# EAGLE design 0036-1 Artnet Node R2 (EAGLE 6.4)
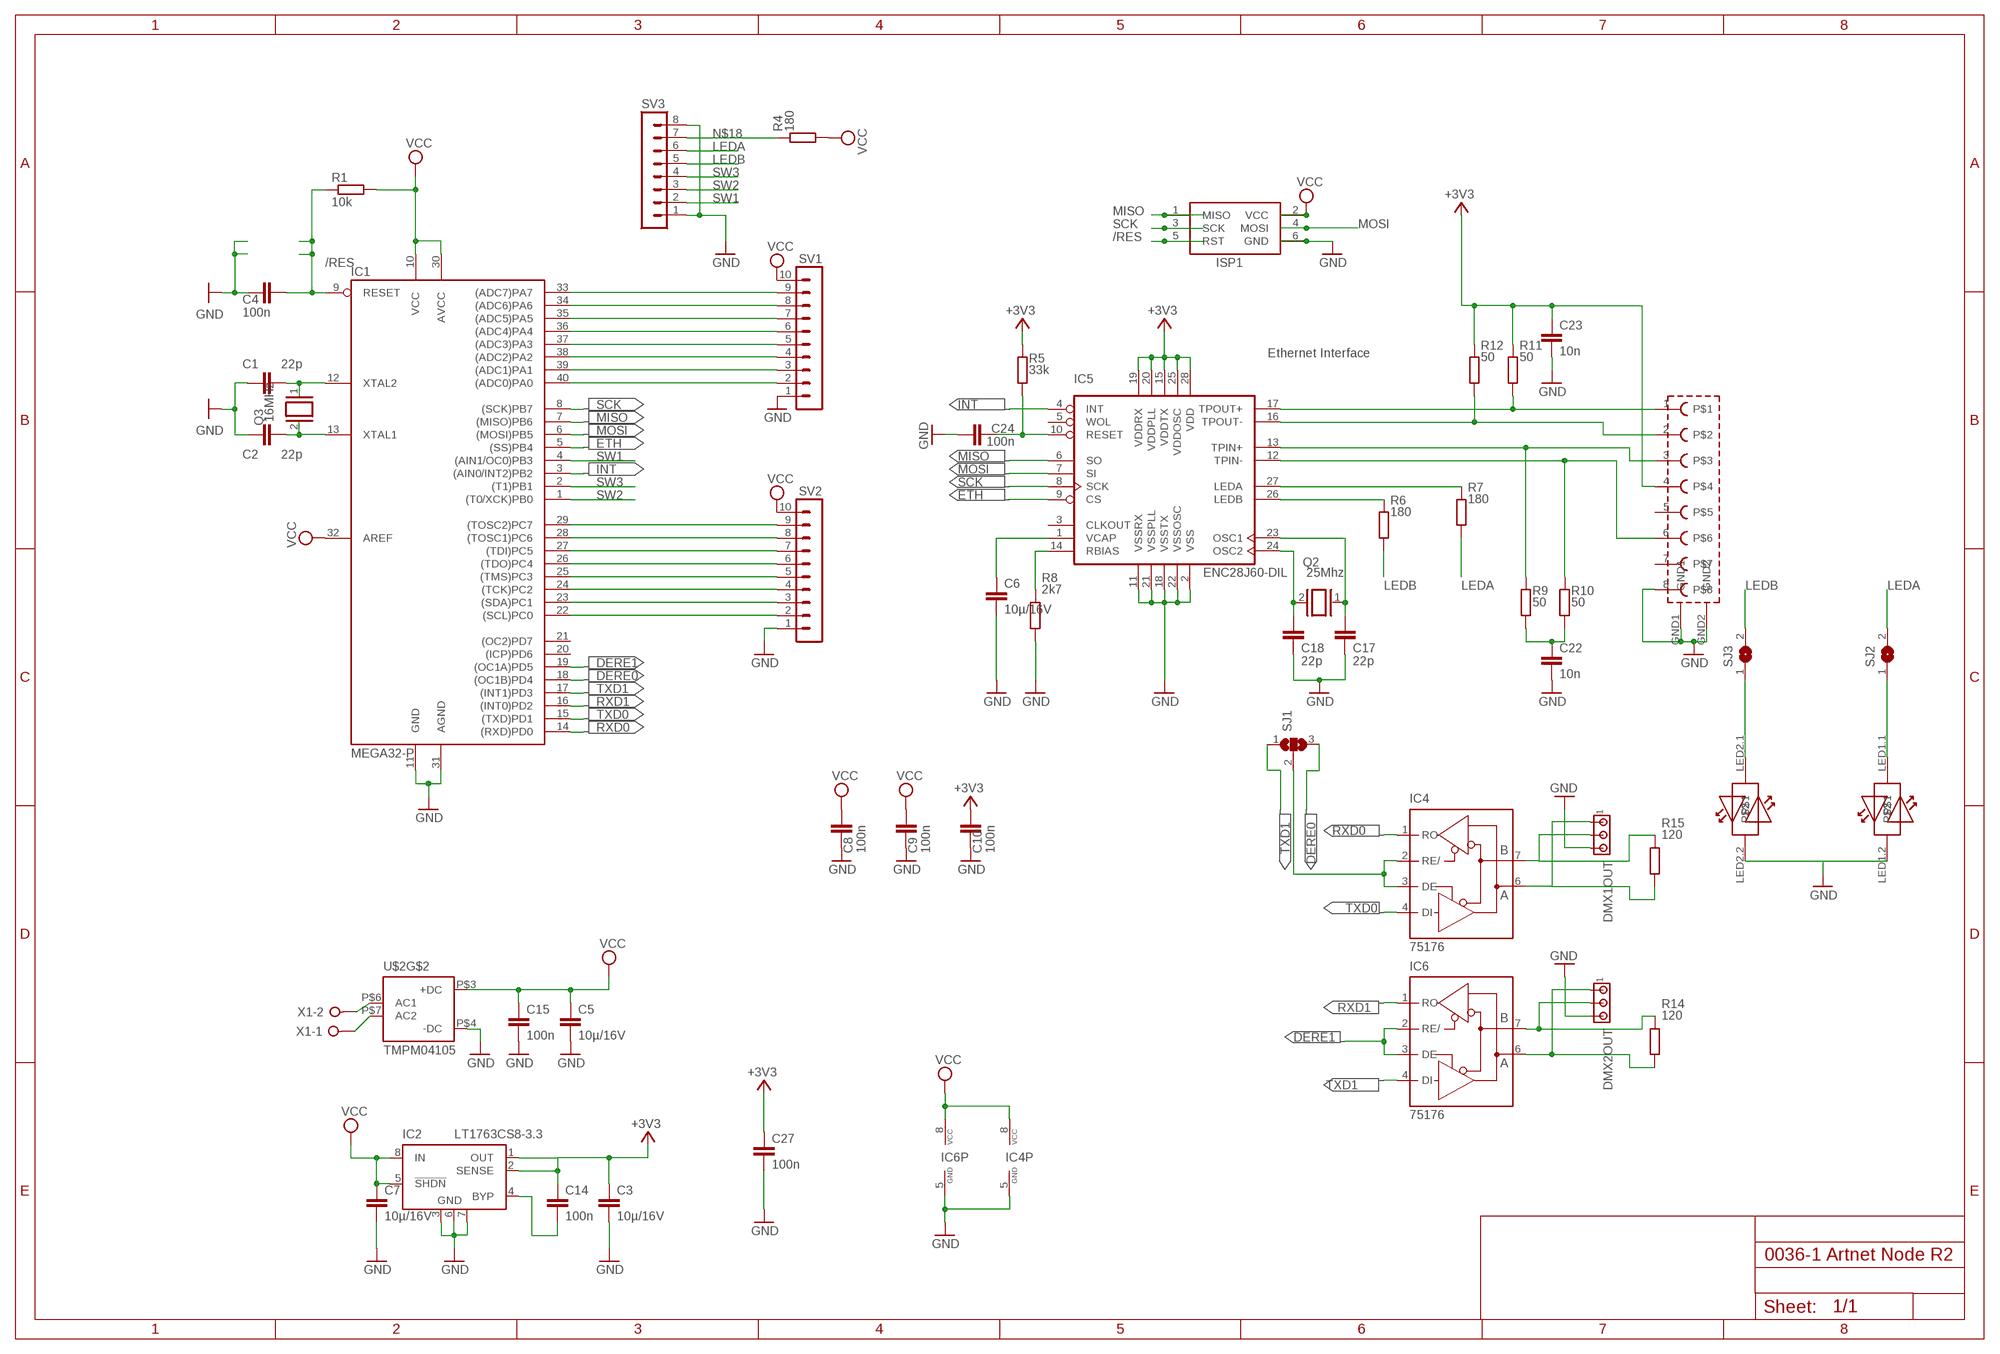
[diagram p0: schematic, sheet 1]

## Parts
C1  22p  C-EUC0805  [C0805]
C2  22p  C-EUC0805  [C0805]
C3  10µ/16V  C-EUC0805  [C0805]
C4  100n  C-EUC0805  [C0805]
C5  10µ/16V  C-EUC0805  [C0805]
C6  10µ/16V  C-EUC0805  [C0805]
C7  10µ/16V  C-EUC0805  [C0805]
C8  100n  C-EUC0805  [C0805]
C9  100n  C-EUC0805  [C0805]
C10  100n  C-EUC0805  [C0805]
C14  100n  C-EUC0805  [C0805]
C15  100n  C-EUC0805  [C0805]
C17  22p  C-EUC0805  [C0805]
C18  22p  C-EUC0805  [C0805]
C22  10n  C-EUC0805  [C0805]
C23  10n  C-EUC0805  [C0805]
C24  100n  C-EUC0805  [C0805]
C27  100n  C-EUC0805  [C0805]
DMX1OUT  MTA03-100  [10X03MTA]
DMX2OUT  MTA03-100  [10X03MTA]
IC1  MEGA32-P  [DIL40]
IC2  LT1763CS8-3.3  [SOIC8]
IC4  75176  MAX481CPA  [DIL08]
IC5  ENC28J60-DIL  [DIL28-3]
IC6  75176  MAX481CPA  [DIL08]
ISP1  AVRISP-6  [AVRISP]
Q2  25Mhz  XTAL/S  [QS]
Q3  16MHz  XTAL/S  [QS]
R1  10k  R-EU_R0805  [R0805]
R4  180  R-EU_R0805  [R0805]
R5  33k  R-EU_R0805  [R0805]
R6  180  R-EU_R0805  [R0805]
R7  180  R-EU_R0805  [R0805]
R8  2k7  R-EU_R0805  [R0805]
R9  50  R-EU_MELF0204W  [MINI_MELF-0204W]
R10  50  R-EU_MELF0204W  [MINI_MELF-0204W]
R11  50  R-EU_MELF0204W  [MINI_MELF-0204W]
R12  50  R-EU_MELF0204W  [MINI_MELF-0204W]
R14  120  R-EU_R0805  [R0805]
R15  120  R-EU_R0805  [R0805]
SJ1  SJ2W  [SJ_2]
SJ2  SJ  [SJ]
SJ3  SJ  [SJ]
SV1  MA10-1  [MA10-1]
SV2  MA10-1  [MA10-1]
SV3  MA08-1  [MA08-1]
U$1  MAGJACK  [MAGJACK]
U$2  TMPM04105  [4WSINGLE]
X1  W237-02P  [W237-132]

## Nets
+3V3: C3.1 C10.2 C14.1 C23.1 C27.1 IC2.1(OUT) IC2.2(SENSE) IC5.15(VDDTX) IC5.19(VDDRX) IC5.20(VDDPLL) IC5.25(VDDOSC) IC5.28(VDD) R5.2 R11.1 R12.1 U$1.4
/RES: C4.2 IC1.9(RESET) ISP1.5(RST) R1.1
DERE0: IC1.18((OC1B)PD4) SJ1.3
DERE1: IC1.19((OC1A)PD5) IC6.2(RE/) IC6.3(DE)
ETH: IC1.5((SS)PB4) IC5.9(CS)
GND: C1.1 C2.1 C3.2 C4.1 C5.2 C6.2 C7.2 C8.1 C9.1 C10.1 C15.2 C17.1 C18.1 C22.2 C23.2 C24.1 C27.2 DMX1OUT.3 DMX2OUT.3 IC1.11(GND) IC1.31(AGND) IC2.3(GND) IC2.6(GND) IC2.7(GND) IC4.5(GND) IC5.2(VSS) IC5.11(VSSRX) IC5.18(VSSTX) IC5.21(VSSPLL) IC5.22(VSSOSC) IC6.5(GND) ISP1.6(GND) R8.1 SV1.1 SV2.1 SV3.1 SV3.8 U$1.8 U$1.GND1 U$1.GND2 U$1.LED1.2 U$1.LED2.2 U$2.P$4(-DC)
INT: IC1.3((AIN0/INT2)PB2) IC5.4(INT)
LEDA: R7.1 SJ2.2 SV3.6
LEDB: R6.1 SJ3.2 SV3.5
MISO: IC1.7((MISO)PB6) IC5.6(SO) ISP1.1(MISO)
MOSI: IC1.6((MOSI)PB5) IC5.7(SI) ISP1.4(MOSI)
N$1: C2.2 IC1.13(XTAL1) Q3.2
N$2: C1.2 IC1.12(XTAL2) Q3.1
N$3: IC4.2(RE/) IC4.3(DE) SJ1.2
N$5: IC1.22((SCL)PC0) SV2.2
N$6: U$2.P$7(AC2) X1.1
N$7: U$2.P$6(AC1) X1.2
N$8: IC1.23((SDA)PC1) SV2.3
N$9: IC1.24((TCK)PC2) SV2.4
N$10: IC1.25((TMS)PC3) SV2.5
N$11: IC5.27(LEDA) R7.2
N$12: IC1.26((TDO)PC4) SV2.6
N$13: IC5.26(LEDB) R6.2
N$14: IC1.27((TDI)PC5) SV2.7
N$15: IC1.28((TOSC1)PC6) SV2.8
N$16: DMX2OUT.1 IC6.6(A) R14.1
N$17: DMX1OUT.1 IC4.6(A) R15.1
N$18: R4.2 SV3.7
N$19: IC1.29((TOSC2)PC7) SV2.9
N$20: C18.2 IC5.24(OSC2) Q2.2
N$21: C17.2 IC5.23(OSC1) Q2.1
N$22: IC5.12(TPIN-) R10.2 U$1.6
N$23: IC5.13(TPIN+) R9.2 U$1.3
N$24: IC5.16(TPOUT-) R12.2 U$1.2
N$25: IC5.17(TPOUT+) R11.2 U$1.1
N$26: IC5.14(RBIAS) R8.2
N$27: C6.1 IC5.1(VCAP)
N$28: SJ3.1 U$1.LED2.1
N$29: C22.1 R9.1 R10.1
N$30: C24.2 IC5.10(RESET) R5.1
N$31: DMX1OUT.2 IC4.7(B) R15.2
N$32: DMX2OUT.2 IC6.7(B) R14.2
N$33: SJ2.1 U$1.LED1.1
N$34: IC1.40((ADC0)PA0) SV1.2
N$35: C14.2 IC2.4(BYP)
N$36: IC1.39((ADC1)PA1) SV1.3
N$37: IC1.38((ADC2)PA2) SV1.4
N$38: IC1.37((ADC3)PA3) SV1.5
N$39: IC1.36((ADC4)PA4) SV1.6
N$40: IC1.35((ADC5)PA5) SV1.7
N$41: IC1.34((ADC6)PA6) SV1.8
N$42: IC1.33((ADC7)PA7) SV1.9
RXD0: IC1.14((RXD)PD0) IC4.1(RO)
RXD1: IC1.16((INT0)PD2) IC6.1(RO)
SCK: IC1.8((SCK)PB7) IC5.8(SCK) ISP1.3(SCK)
SW1: IC1.4((AIN1/OC0)PB3) SV3.2
SW2: IC1.1((T0/XCK)PB0) SV3.3
SW3: IC1.2((T1)PB1) SV3.4
TXD0: IC1.15((TXD)PD1) IC4.4(DI)
TXD1: IC1.17((INT1)PD3) IC6.4(DI) SJ1.1
VCC: C5.1 C7.1 C8.2 C9.2 C15.1 IC1.10(VCC) IC1.30(AVCC) IC1.32(AREF) IC2.5(!SHDN) IC2.8(IN) IC4.8(VCC) IC6.8(VCC) ISP1.2(VCC) R1.2 R4.1 SV1.10 SV2.10 U$2.P$3(+DC)
Unconnected: IC1.20((ICP)PD6) IC1.21((OC2)PD7) IC5.3(CLKOUT) IC5.5(WOL) U$1.5 U$1.7

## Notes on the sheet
- Ethernet Interface

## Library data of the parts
C1-C10 C14 C15 C17 C18 C22-C24 C27 = rcl:C-EU: CAPACITOR, European symbol
DMX1OUT DMX2OUT = con-amp:MTA03-100: AMP connector
IC1 = avr-1:MEGA32-P: MICROCONTROLLER 32 Kbytes FLASH 2 Kbytes SRAM 1 Kbytes EEPROM USART 8-channel 10 bit ADC
IC2 = linear-technology:LT1763CS8: 500mA, Low Noise, LDO Micropower Regulators Source: http://cds.linear.com/docs/Datasheet/1763ff.pdf; MPN: LT1763CS8-3.3; OC_FARNELL: 1273617; OC_NEWARK: 57M6055
IC4 IC6 = maxim:MAX481CPA: RS485 TRANSEIVER; MPN: MAX481CPA+; OC_FARNELL: unknown; OC_NEWARK: 99K3445
IC5 = enc28j60centered:ENC28J60-*: Microchip 10Mbit Ethernet controller with SPI interface Improved SOIC28 layout (pads in 0.01 raster, pin1 slightly smaller). Pin 6 (SO) changed from Out (paralleling several Outs gives an error) to OC. Author: Profi from mikrocontroller.net - forum Date: 2006.0827
ISP1 = adafruit:AVRISP: AVR ISP HEADER Standard 6 pin header for AVR programming
Q2 Q3 = special:XTAL/S: CRYSTAL
R1 R4-R12 R14 R15 = rcl:R-EU_: RESISTOR, European symbol
SJ1 = jumper:SJ2W: SMD solder JUMPER
SJ2 SJ3 = jumper:SJ: SMD solder JUMPER
SV1 SV2 = con-lstb:MA10-1: PIN HEADER; OC_FARNELL: unknown; OC_NEWARK: unknown
SV3 = con-lstb:MA08-1: PIN HEADER; OC_FARNELL: unknown; OC_NEWARK: unknown
U$1 = magjacksmalldrill:MAGJACK
U$2 = TRACO ACDC:TMPM04105
X1 = con-wago-508:W237-02P: WAGO SREW CLAMP; OC_FARNELL: unknown; OC_NEWARK: unknown

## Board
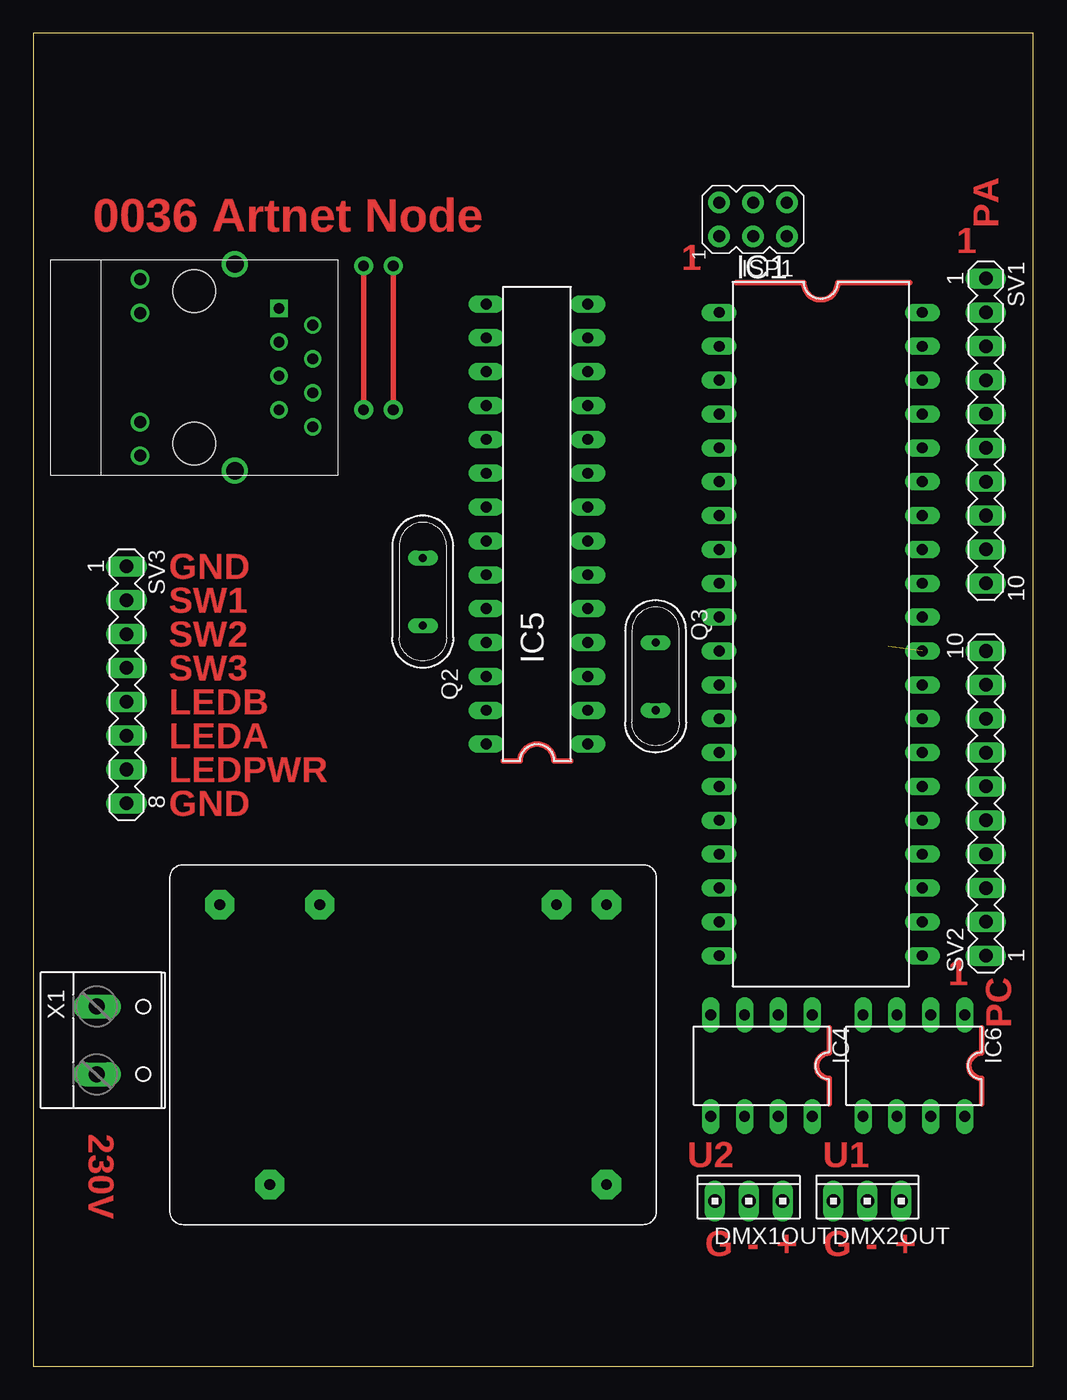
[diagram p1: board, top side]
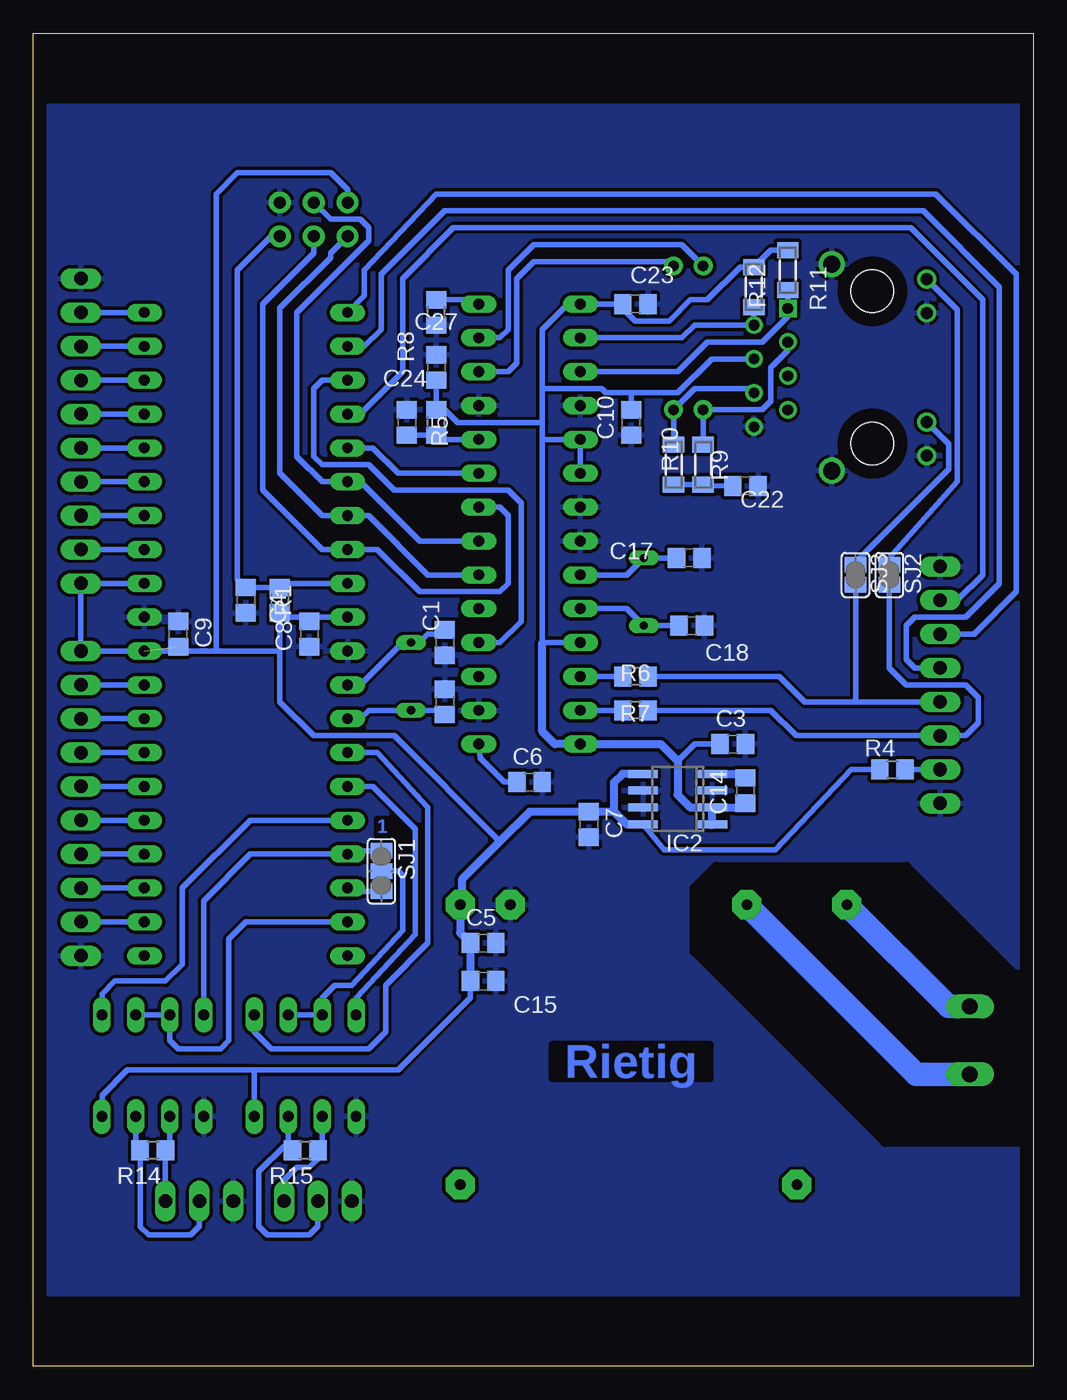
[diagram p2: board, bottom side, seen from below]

Size 75 x 100 mm. Coordinates in mm from the lower left corner, seen from the top.
Outline: 0,0 75,0 75,100 0,100 0,0
Copper layers (1*16): Top 0.035mm / dielectric 1.5mm / Bottom 0.035mm
Design rules "default": minimum track width 10mil, minimum drill 24mil, track to track 8mil, track to pad 8mil, pad to pad 8mil, via to via 8mil, smd to smd 8mil, copper to edge 40mil, drill to drill 8mil, minimum pad ring 10mil, minimum via ring 8mil, stop-mask expansion 4mil, vias tented up to drill 0mil, thermal gap 10mil
bRestrict: area 0,16.8 to 25.4,37.5; area 0,95 to 75,100; area 0,0 to 75,5

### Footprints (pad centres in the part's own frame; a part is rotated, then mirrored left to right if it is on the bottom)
C0805 = smd 1.3 x 1.5: 1 -0.95,0; 2 0.95,0
10X03MTA = drill 1.016 long: 1 2.54,0; 2 0,0; 3 -2.54,0
DIL40 = drill 0.813 long: 1 -24.13,-7.62; 2 -21.59,-7.62; 3 -19.05,-7.62; 4 -16.51,-7.62; 5 -13.97,-7.62; 6 -11.43,-7.62; 7 -8.89,-7.62; 8 -6.35,-7.62; 9 -3.81,-7.62; 10 -1.27,-7.62; 11 1.27,-7.62; 12 3.81,-7.62; 13 6.35,-7.62; 14 8.89,-7.62; 15 11.43,-7.62; 16 13.97,-7.62; 17 16.51,-7.62; 18 19.05,-7.62; 19 21.59,-7.62; 20 24.13,-7.62; 21 24.13,7.62; 22 21.59,7.62; 23 19.05,7.62; 24 16.51,7.62; 25 13.97,7.62; 26 11.43,7.62; 27 8.89,7.62; 28 6.35,7.62; 29 3.81,7.62; 30 1.27,7.62; 31 -1.27,7.62; 32 -3.81,7.62; 33 -6.35,7.62; 34 -8.89,7.62; 35 -11.43,7.62; 36 -13.97,7.62; 37 -16.51,7.62; 38 -19.05,7.62; 39 -21.59,7.62; 40 -24.13,7.62
SOIC8 = smd 0.6 x 2.2: 1 -1.905,-2.6; 2 -0.635,-2.6; 3 0.635,-2.6; 4 1.905,-2.6; 5 1.905,2.6; 6 0.635,2.6; 7 -0.635,2.6; 8 -1.905,2.6
DIL08 = drill 0.813 long: 1 -3.81,-3.81; 2 -1.27,-3.81; 3 1.27,-3.81; 4 3.81,-3.81; 5 3.81,3.81; 6 1.27,3.81; 7 -1.27,3.81; 8 -3.81,3.81
DIL28-3 = drill 0.813 long: 1 -16.51,-3.81; 2 -13.97,-3.81; 3 -11.43,-3.81; 4 -8.89,-3.81; 5 -6.35,-3.81; 6 -3.81,-3.81; 7 -1.27,-3.81; 8 1.27,-3.81; 9 3.81,-3.81; 10 6.35,-3.81; 11 8.89,-3.81; 12 11.43,-3.81; 13 13.97,-3.81; 14 16.51,-3.81; 15 16.51,3.81; 16 13.97,3.81; 17 11.43,3.81; 18 8.89,3.81; 19 6.35,3.81; 20 3.81,3.81; 21 1.27,3.81; 22 -1.27,3.81; 23 -3.81,3.81; 24 -6.35,3.81; 25 -8.89,3.81; 26 -11.43,3.81; 27 -13.97,3.81; 28 -16.51,3.81
AVRISP = drill 0.9 pad 1.626: 1 -1.27,2.54; 2 1.27,2.54; 3 -1.27,0; 4 1.27,0; 5 -1.27,-2.54; 6 1.27,-2.54
QS = drill 0.61 long: 1 -2.54,0; 2 2.54,0
R0805 = smd 1.3 x 1.5: 1 -0.95,0; 2 0.95,0
MINI_MELF-0204W = smd 1.2 x 1.6: 1 -1.5,0; 2 1.5,0
SJ_2 = smd 1.168 x 1.6: 1 -1.524,0; 2 0,0; 3 1.524,0
SJ = smd 1.168 x 1.6: 1 -0.762,0; 2 0.762,0
MA10-1 = drill 1.016 long: 1 -11.43,0; 2 -8.89,0; 3 -6.35,0; 4 -3.81,0; 5 -1.27,0; 6 1.27,0; 7 3.81,0; 8 6.35,0; 9 8.89,0; 10 11.43,0
MA08-1 = drill 1.016 long: 1 -8.89,0; 2 -6.35,0; 3 -3.81,0; 4 -1.27,0; 5 1.27,0; 6 3.81,0; 7 6.35,0; 8 8.89,0
MAGJACK = drill 0.8 square: 1 -4.445,6.35 | drill 0.8: 2 -3.175,8.89; 3 -1.905,6.35; 4 -0.635,8.89; 5 0.635,6.35; 6 1.905,8.89; 7 3.175,6.35; 8 4.445,8.89 | drill 1.3: GND1 -7.747,3.048; GND2 7.747,3.048 | drill 0.9: LED1.1 -6.629,-4.064; LED1.2 -4.089,-4.064; LED2.1 4.089,-4.064; LED2.2 6.629,-4.064 | hole 3.2: -5.715,0; 5.715,0
4WSINGLE = drill 0.8 pad 2.184 octagon: P$1 10.823,-10.206; P$2 10.823,15.044; P$3 -10.177,15.044; P$4 -10.177,11.294; P$6 -10.177,-6.455; P$7 -10.177,-13.956
W237-132 = drill 1.194 long: 1 -2.54,-0.635; 2 2.54,-0.635

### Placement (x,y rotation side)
C1  44.13,54.29 90 bottom
C2  44.13,49.85 270 bottom
C3  22.54,46.67 0 bottom
C4  59.05,57.47 90 bottom
C5  41.27,31.75 0 bottom
C6  37.78,43.81 0 bottom
C7  33.34,40.64 270 bottom
C8  54.29,54.93 90 bottom
C9  64.14,54.93 270 bottom
C10  30.16,70.8 90 bottom
C14  21.59,43.18 90 bottom
C15  41.27,28.89 0 bottom
C17  25.81,60.64 180 bottom
C18  25.62,55.56 180 bottom
C22  21.59,66.04 0 bottom
C23  29.84,79.69 0 bottom
C24  46.99,70.8 270 bottom
C27  44.77,74.93 90 bottom
DMX1OUT  53.66,12.38 0 top
DMX2OUT  62.55,12.38 0 top
IC1  59.05,54.93 270 top
IC2  26.67,42.55 90 bottom
IC4  54.61,22.54 180 top
IC5  37.78,63.18 90 top
IC6  66.04,22.54 180 top
ISP1  53.98,86.04 90 top
Q2  29.21,58.1 270 top
Q3  46.67,51.75 270 top
R1  56.52,57.47 270 bottom
R4  10.57,44.77 0 bottom
R5  44.77,70.8 90 bottom
R6  29.84,51.75 180 bottom
R7  29.84,49.21 180 bottom
R8  44.77,79.06 90 bottom
R9  24.77,67.63 90 bottom
R10  26.99,67.63 90 bottom
R11  18.41,82.23 270 bottom
R12  20.95,80.96 270 bottom
R14  66.04,16.19 180 bottom
R15  54.61,16.19 180 bottom
SJ1  48.9,37.15 270 bottom
SJ2  10.79,59.37 270 bottom
SJ3  13.34,59.37 270 bottom
SV1  71.44,70.17 270 top
SV2  71.44,42.23 90 top
SV3  6.99,51.12 270 top
U$1  12.06,74.93 270 top
U$2  27.94,24.45 270 top
X1  5.4,24.45 270 top

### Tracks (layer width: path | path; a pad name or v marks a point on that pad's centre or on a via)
+3V3
  Bottom 0.406: IC5.25 36.83,54.29 36.83,69.53 | IC5.20 IC5.19 | C27.1 44.77,72.07 R5.2 44.13,71.75 43.18,70.8 36.83,70.8 | 36.83,69.53 36.83,70.8 | 36.83,70.8 36.83,73.34 | 36.83,73.34 36.83,77.79 34.92,79.69 IC5.15 C23.1 30.48,79.38 30.48,79.06 29.84,78.42 27.3,78.42 25.72,80.01 24.45,80.01 22,82.46 R12.1 19.68,83.73 R11.1 | IC5.19 36.83,69.53 | C3.1 25.4,46.67 26.67,45.4 | U$1.4 24.13,75.56 26.67,73.03 30.16,73.03 | 33.66,69.22 IC5.19 | 30.16,73.03 32.07,73.03 32.38,73.34 36.83,73.34 | C10.2 30.16,73.03
  Bottom 0.61: 36.83,54.29 36.83,47.62 35.88,46.67 IC5.28 27.94,46.67 26.67,45.4 26.67,42.86 25.72,41.91 IC2.2 | IC2.2 21.59,41.91 C14.1 | 24.13,40.58 IC2.1 IC2.2
+6874
  Top 0.406: 60.33,81.28 arc-180 57.78,81.28 52.7,81.28
/RES
  Bottom 0.406: IC1.9 56.2,58.74 R1.1 C4.2 59.69,59.05 59.69,82.23 57.15,84.77 ISP1.5
DERE0
  Bottom 0.406: SJ1.3 51.18,35.62 IC1.18
DERE1
  Bottom 0.406: IC6.2 IC6.3 64.77,24.45 64.14,23.81 60.96,23.81 60.33,24.45 60.33,32.07 59.05,33.34 IC1.19
ETH
  Bottom 0.406: IC5.9 47.62,66.99 49.53,68.9 IC1.5
GND
  pour Bottom (isolate 0.254, rank 6): -0.84,101.07 -3.48,-6.05 78.42,-5.65 79.07,101.2
INT
  Bottom 0.406: IC5.4 40.01,54.29 38.42,55.88 38.42,64.77 39.37,65.72 47.94,65.72 49.85,67.63 53.34,67.63 53.98,68.26 53.98,73.34 53.34,73.98 IC1.3
LEDA
  Bottom 0.406: R7.1 19.68,49.21 17.78,47.31 SV3.6 5.08,47.31 4.13,48.26 4.13,50.16 5.08,51.12 9.53,51.12 10.79,52.39 SJ2.2
LEDB
  Bottom 0.406: R6.1 19.05,51.75 17.14,49.85 13.34,49.85 | 13.34,49.85 SV3.5 | SJ3.2 13.34,49.85
MISO
  Bottom 0.406: IC5.6 45.4,59.37 49.85,63.82 IC1.7 53.34,63.82 56.52,66.99 56.52,79.38 52.7,83.19 52.7,83.5 ISP1.1
MOSI
  Bottom 0.406: IC5.7 46.04,61.91 50.48,66.36 IC1.6 53.34,66.36 55.24,68.26 55.24,79.06 49.85,84.45 49.85,85.41 50.48,86.04 52.7,86.04 ISP1.4
N$1
  Bottom 0.406: IC1.13 50.48,48.58 49.85,49.21 Q3.2 44.45,49.21 C2.2
N$2
  Bottom 0.406: IC1.12 50.48,51.12 47.31,54.29 Q3.1 46.04,54.29 45.4,54.93 44.45,54.93 C1.2
N$3
  Bottom 0.406: IC4.2 IC4.3 53.34,27.62 52.39,28.57 51.12,28.57 47.31,32.7 47.31,36.83 47.62,37.15 SJ1.2
N$5
  Bottom 0.406: IC1.22 SV2.2
N$6
  Bottom 1.778: X1.1 6.35,26.99 U$2.P$7
N$7
  Bottom 1.778: X1.2 8.77,21.91 U$2.P$6
N$8
  Bottom 0.406: IC1.23 SV2.3
N$9
  Bottom 0.406: IC1.24 SV2.4
N$10
  Bottom 0.406: IC1.25 SV2.5
N$11
  Bottom 0.406: IC5.27 R7.2
N$12
  Bottom 0.406: IC1.26 SV2.6
N$13
  Bottom 0.406: R6.2 IC5.26
N$14
  Bottom 0.406: IC1.27 SV2.7
N$15
  Bottom 0.406: IC1.28 SV2.8
N$16
  Bottom 0.406: IC6.6 64.77,16.51 R14.1 DMX2OUT.1
N$17
  Bottom 0.406: IC4.6 53.34,16.2 | 53.34,16.2 R15.1 | 53.34,16.2 53.34,15.88 54.29,14.92 55.24,14.92 56.2,13.97 DMX1OUT.1
N$18
  Bottom 0.406: SV3.7 R4.2
N$19
  Bottom 0.406: IC1.29 SV2.9
N$20
  Bottom 0.406: IC5.24 30.48,56.83 Q2.2 C18.2
N$21
  Bottom 0.406: IC5.23 30.48,59.37 Q2.1 C17.2
N$22  (via drill 0.8 pad 1.42)
  Top 0.406: v26.99,71.75 v26.99,82.55
  Bottom 0.406: IC5.12 39.37,74.61 38.73,75.25 38.73,81.6 37.47,82.87 27.3,82.87 v26.99,82.55 | R10.2 v26.99,71.75 25.4,73.34 21.27,73.34 U$1.6
N$23  (via drill 0.8 pad 1.42)
  Top 0.406: v24.77,82.55 v24.77,71.75
  Bottom 0.406: v24.77,82.55 26.35,84.14 37.47,84.14 39.37,82.23 39.37,77.79 40.01,77.15 IC5.13 | R9.2 v24.77,71.75 20.32,71.75 19.68,72.39 19.68,74.93 18.41,76.2 U$1.3
N$24
  Bottom 0.406: IC5.16 26.35,77.15 25.4,78.11 U$1.2 R12.2
N$25
  Bottom 0.406: IC5.17 26.67,74.61 24.45,76.83 20.32,76.83 18.41,78.74 U$1.1 R11.2
N$26
  Bottom 0.406: R8.2 41.81,80.01 IC5.14
N$27
  Bottom 0.406: IC5.1 41.5,45.63 39.69,43.81 C6.1
N$28
  Bottom 0.406: SJ3.1 13.34,60.33 6.35,67.31 6.35,69.19 U$1.LED2.1
N$29
  Bottom 0.406: R9.1 R10.1 C22.1
N$30
  Bottom 0.406: IC5.10 44.77,69.53 R5.1 C24.2
N$31
  Bottom 0.406: IC4.7 55.88,16.2 R15.2 56.2,16.51 58.1,14.61 58.1,10.48 57.47,9.84 54.29,9.84 53.66,10.48 DMX1OUT.2
N$32
  Bottom 0.406: IC6.7 67.31,16.51 R14.2 66.99,10.47 66.36,9.84 63.18,9.84 62.55,10.48 DMX2OUT.2
N$33
  Bottom 0.406: SJ2.1 10.79,60.64 5.71,66.36 5.71,79.27 U$1.LED1.1
N$34
  Bottom 0.406: IC1.40 SV1.2
N$35
  Bottom 0.61: IC2.4 21.59,44.45 C14.2
N$36
  Bottom 0.406: IC1.39 SV1.3
N$37
  Bottom 0.406: IC1.38 SV1.4
N$38
  Bottom 0.406: IC1.37 SV1.5
N$39
  Bottom 0.406: IC1.36 SV1.6
N$40
  Bottom 0.406: IC1.35 SV1.7
N$41
  Bottom 0.406: IC1.34 SV1.8
N$42
  Bottom 0.406: IC1.33 SV1.9
N$43
  Top 0.406: 59.69,19.68 59.69,21.59 arc-180 59.69,23.5 59.69,25.4
N$44
  Top 0.406: 60.33,81.28 65.72,81.28
N$45
  Top 0.406: 35.24,45.4 36.51,45.4 arc-180 39.05,45.4 40.32,45.4
N$47
  Top 0.406: 71.12,23.5 71.12,25.4
N$4654
  Top 0.406: 71.12,23.5 arc180 71.12,21.59 71.12,19.68
RXD0
  Bottom 0.406: IC4.1 58.42,25.08 57.15,23.81 49.85,23.81 48.58,25.08 48.58,28.57 45.4,31.75 45.4,41.91 49.21,46.04 IC1.14
RXD1
  Bottom 0.406: IC1.16 58.74,40.96 63.82,35.88 63.82,30.16 65.09,28.89 68.9,28.89 69.85,27.94 IC6.1
SCK
  Bottom 0.406: IC5.8 40.01,64.45 39.37,63.82 39.37,58.74 40.01,58.1 46.04,58.1 49.21,61.28 IC1.8 53.34,61.28 57.78,65.72 57.78,79.69 53.98,83.5 ISP1.3
SW1
  Bottom 0.406: IC1.4 50.48,71.44 47.31,74.61 47.31,81.6 43.5,85.41 9.21,85.41 3.81,80.01 3.81,59.37 5.71,57.47 SV3.2
SW2
  Bottom 0.406: SV3.3 4.45,54.93 1.27,58.1 1.27,81.92 7.3,87.95 44.77,87.95 50.16,82.23 50.16,80.33 IC1.1
SW3
  Bottom 0.406: SV3.4 8.89,52.39 9.53,53.02 9.53,55.56 8.89,56.2 5.08,56.2 2.54,58.74 2.54,80.96 8.26,86.68 44.13,86.68 48.9,81.92 48.9,77.79 50.16,76.52 IC1.2
TXD0
  Bottom 0.406: IC1.15 49.53,43.5 46.35,40.32 46.35,32.38 50.8,27.62 IC4.4
TXD1
  Bottom 0.406: IC6.4 62.23,34.92 58.74,38.42 IC1.17 51.18,38.67 SJ1.1
VCC  (1 unrouted)
  Bottom 0.406: IC1.10 54.29,56.2 | 54.29,56.2 56.52,56.2 | 56.52,56.2 56.52,53.66 | 56.52,53.66 56.52,49.85 53.98,47.31 47.94,47.31 40.01,39.37 | 58.42,22.23 | IC4.8 58.42,22.23 | 58.42,22.23 67.94,22.23 69.85,20.32 IC6.8 | R4.1 13.65,44.77 19.37,38.73 27.68,38.73 IC2.8 | 31.43,41.59 31.43,43.81 | IC1.32 SV1.10 SV2.10 IC1.30 61.28,53.66 | R1.2 56.52,56.2 | 56.52,53.66 61.28,53.66 | 58.42,22.23 47.62,22.23 42.23,27.62 C15.1 | ISP1.2 51.44,88.27 52.7,89.53 59.69,89.53 61.28,87.95 61.28,53.66 | C8.2 54.29,56.2
  Bottom 0.61: IC2.5 30.8,44.45 31.43,43.81 31.43,41.59 30.48,40.64 IC2.8 | 31.43,41.59 C7.1 37.78,41.59 40.01,39.37 42.86,36.51 42.86,34.75 U$2.P$3 42.98,32.51 C5.1 C15.1

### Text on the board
Top: PA | 0036 Artnet Node | 1 | 1 | GND | SW1 | SW2 | SW3 | LEDB | LEDA | LEDPWR | GND | 1 | PC | 230V | U2 | U1 | G | - | + | G | - | +
Bottom: 1 | Rietig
